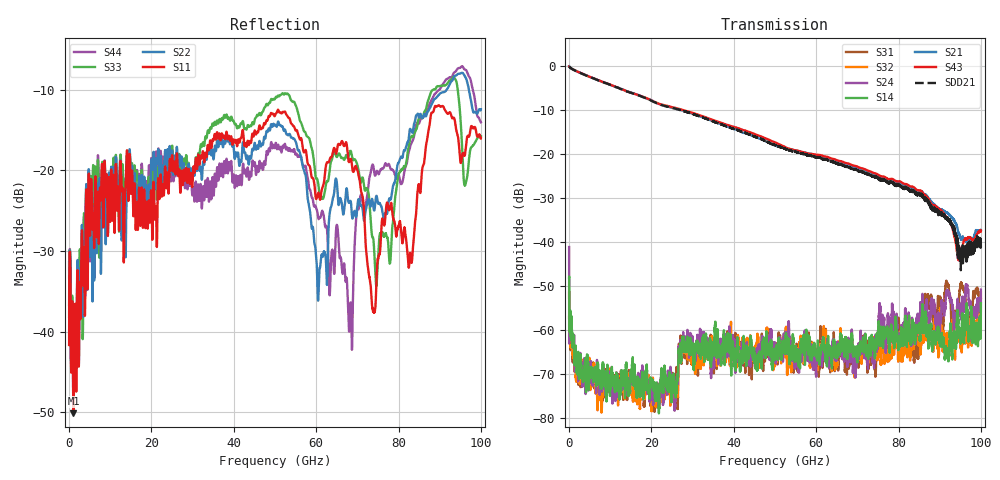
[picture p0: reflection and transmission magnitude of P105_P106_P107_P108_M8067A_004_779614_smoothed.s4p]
!Keysight Technologies PLTS 2021(64 bit), Build 20210202.1
!S11 smoothed in format LOGMAG, average points = 21
!S12 smoothed in format LOGMAG, average points = 21
!S13 smoothed in format LOGMAG, average points = 21
!S14 smoothed in format LOGMAG, average points = 21
!S21 smoothed in format LOGMAG, average points = 21
!S22 smoothed in format LOGMAG, average points = 21
!S23 smoothed in format LOGMAG, average points = 21
!S24 smoothed in format LOGMAG, average points = 21
!S31 smoothed in format LOGMAG, average points = 21
!S32 smoothed in format LOGMAG, average points = 21
!S33 smoothed in format LOGMAG, average points = 21
!S34 smoothed in format LOGMAG, average points = 21
!S41 smoothed in format LOGMAG, average points = 21
!S42 smoothed in format LOGMAG, average points = 21
!S43 smoothed in format LOGMAG, average points = 21
!S44 smoothed in format LOGMAG, average points = 21
!$DUT_CFG_DESC: Default 4-Port Configuration
!$NUMBER_PORTS: 4
!$DIFF_PORT_MAP: 1|2P|2|2P|0|UC|0|UC|
!$PORT_MAP: 1|1|<<<<<<|2|2|>>>>>>|3|3|<<<<<<|4|4|>>>>>>|
!Date: Monday, December 04, 2023, 05:51:54
!S4P File: Measurements: <S11,S12,S13,S14>,
!<S21,S22,S23,S24>,
!<S31,S32,S33,S34>,
!<S41,S42,S43,S44>:
# MHz S  RI  R 50
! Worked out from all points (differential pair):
!   10000 points, 10 MHz to 100 GHz, reference 50 ohm
!   strongest paths, dB at 10 MHz, 25.01 GHz, 50.01 GHz, 75.01 GHz, 100 GHz:
!     S43: -0.2, -9.4, -17.4, -24.7, -37.5
!     S21: -0.1, -9.5, -18.1, -25.0, -37.4
!     S14: -48.1, -73.3, -66.6, -61.6, -54.0
!     S24: -41.2, -73.6, -64.7, -60.4, -50.9
!     S32: -57.2, -75.9, -67.4, -64.7, -51.5
!     S31: -52.7, -71.8, -64.7, -65.6, -52.8
!   taken as a pair (ports 3,1 in; 4,2 out), SDD21 dB: -0.1, -9.6, -18.0, -25.5, -41.3
!   lowest |S11| = -50.1 dB at 1.05 GHz (marker M1), VSWR 1.01, Z = 50.2 + j0.271 ohm
!   |S11| at or under -10 dB: start of sweep to end of sweep
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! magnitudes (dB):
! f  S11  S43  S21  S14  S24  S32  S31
! 10 MHz  -41.7  -0.2  -0.1  -48.1  -41.2  -57.2  -52.7
! 1.05 GHz  -50.1  -0.9  -0.9  -62.7  -63.1  -64.9  -66.7
! 14.42 GHz  -23.6  -5.9  -5.9  -74.5  -75.0  -73.1  -70.8
! 54.4 GHz  -14.5  -19.1  -19.1  -62.3  -65.0  -66.8  -68.9
! 68.34 GHz  -18.6  -22.4  -22.9  -64.1  -66.3  -66.5  -67.0
! 73.98 GHz  -37.5  -24.4  -24.7  -64.5  -65.4  -63.4  -66.0
! 100 GHz  -16.0  -37.5  -37.4  -54.0  -50.9  -51.5  -52.8
